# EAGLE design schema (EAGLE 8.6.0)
CNAME: Garden light controller with hysteresis; CREVISION: 4; CVERSION: V 1.0; DATECODE: 8/07/2017; DESIGNER: Michy
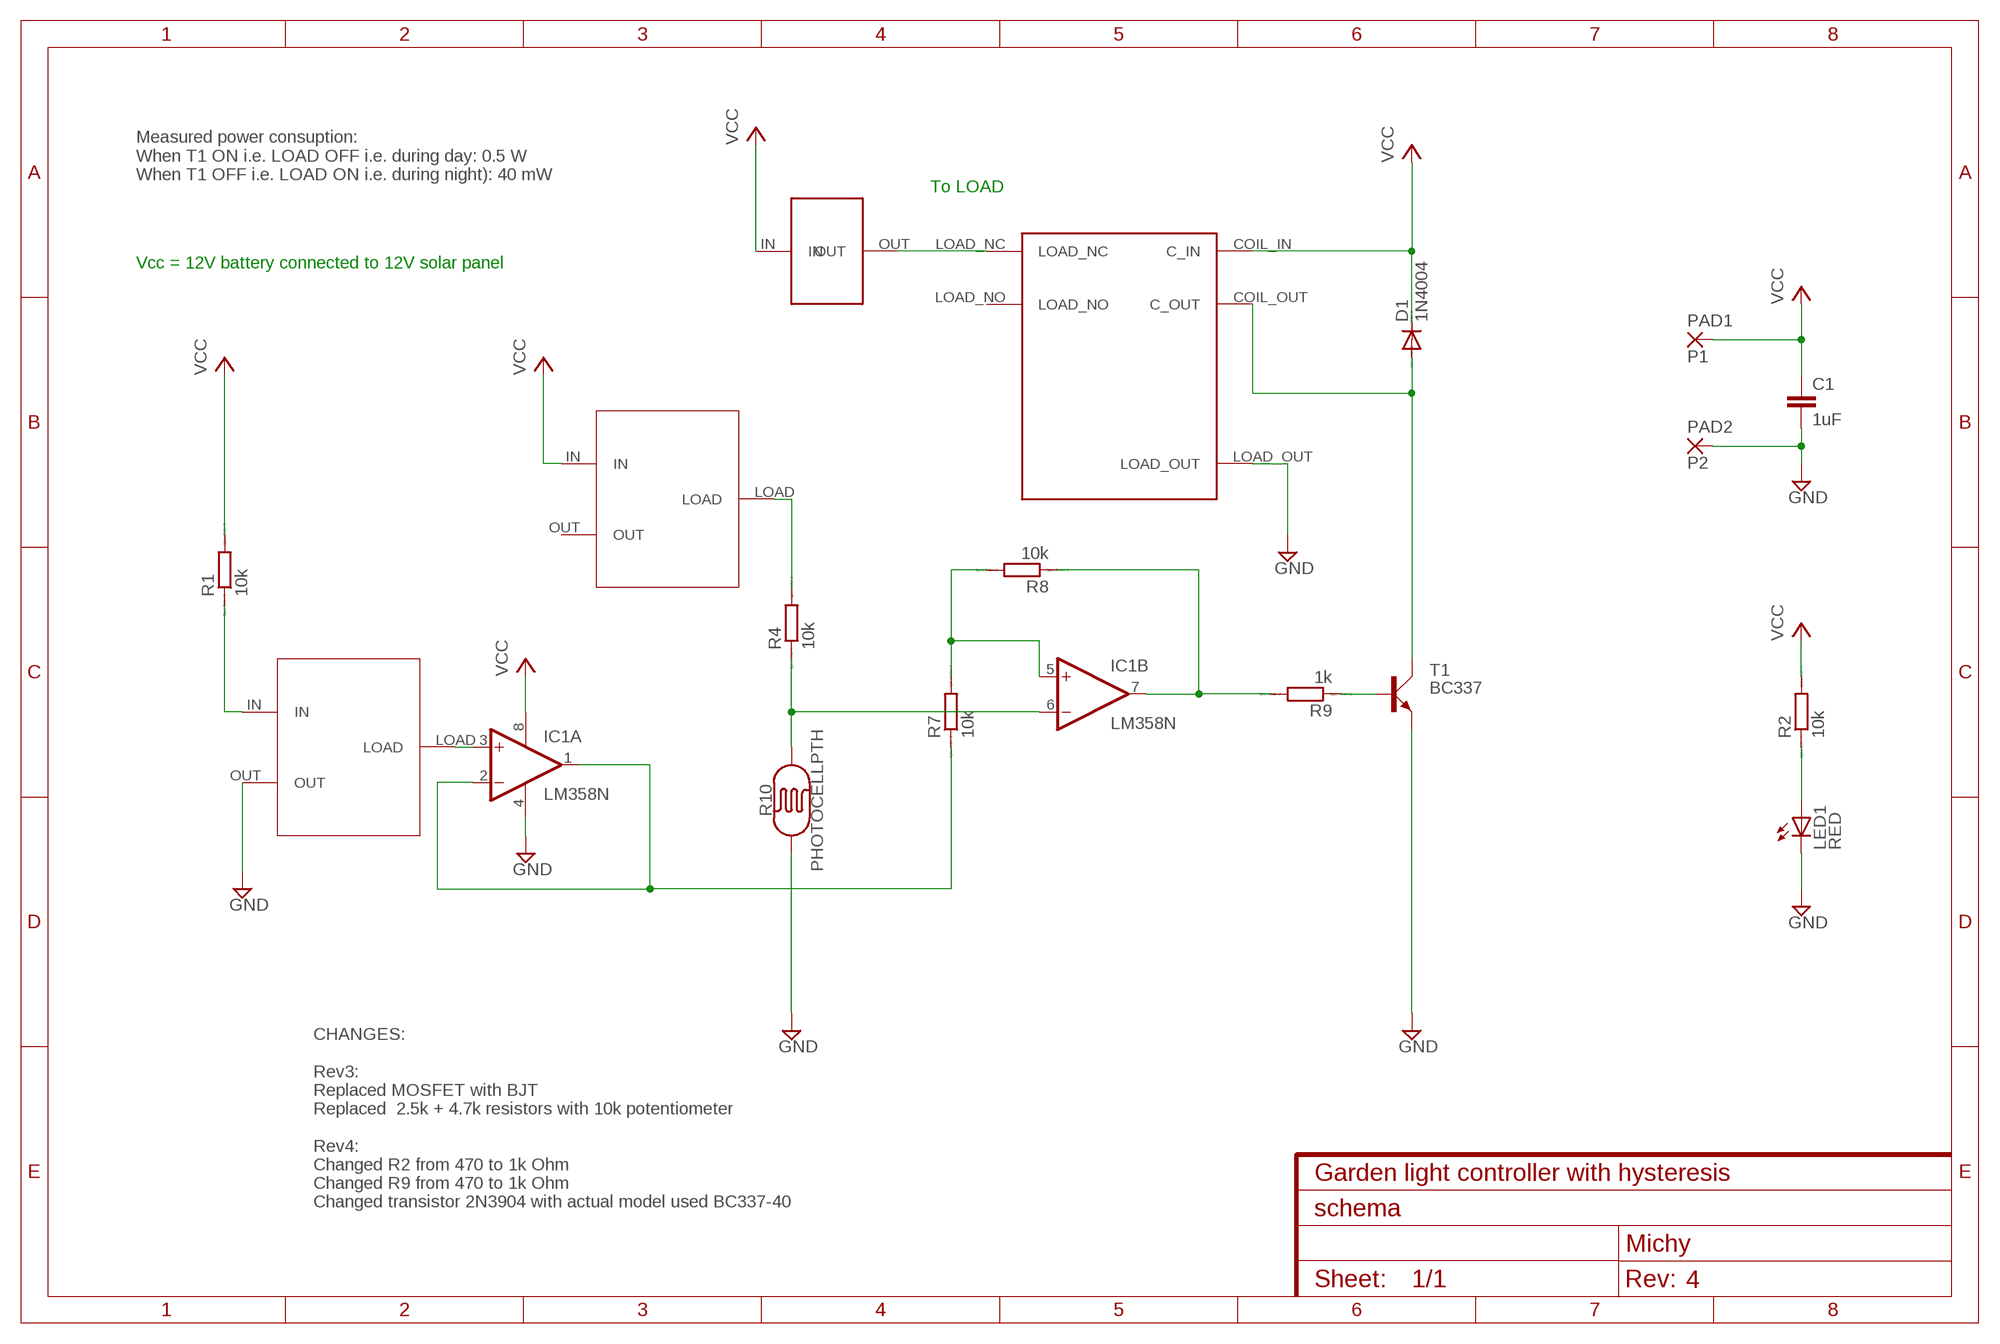
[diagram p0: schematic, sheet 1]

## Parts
C1  1uF  C-EU025-025X050  [C025-025X050]
D1  1N4004  [DO41-10]
IC1  LM358N  [DIL08]
LED1  RED  LED3MM  [LED3MM]
PAD1  P1  1,6/0,8  [1,6/0,8]
PAD2  P2  1,6/0,8  [1,6/0,8]
R1  10k  R0207/10  [0207/10]
R2  10k  R0207/10  [0207/10]
R4  10k  R0207/10  [0207/10]
R7  10k  R0207/10  [0207/10]
R8  10k  R0207/10  [0207/10]
R9  1k  R0207/10  [0207/10]
R10  PHOTOCELLPTH  [PHOTOCELL]
T1  BC337  [SOT54A]
U$1  SRSZ-12VDC-SL  [SRSZ-12VDC-SL]
U$2  ACPSPAIN22K  [ACPSPAIN22K]
U$3  ACPSPAIN22K  [ACPSPAIN22K]
U$4  DEVICEOUTLET  [OUTLET]

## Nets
GND: C1.2 IC1.4(P:V-) LED1.K(C) PAD2.1(P) R10.1 T1.E U$1.LOAD_OUT U$2.OUT
N$1: R1.1 U$2.IN
N$2: IC1.1(A:OUT) IC1.2(A:-IN) R7.1
N$3: R9.1 T1.B
N$4: LED1.A R2.1
N$5: IC1.6(B:-IN) R4.1 R10.2
N$6: R4.2 U$3.LOAD
N$7: IC1.7(B:OUT) R8.1 R9.2
N$8: IC1.5(B:+IN) R7.2 R8.2
N$9: D1.A T1.C U$1.COIL_OUT(C_OUT)
N$10: IC1.3(A:+IN) U$2.LOAD
N$11: U$1.LOAD_NC U$4.OUT
VCC: C1.1 D1.C IC1.8(P:V+) PAD1.1(P) R1.2 R2.2 U$1.COIL_IN(C_IN) U$3.IN U$4.IN
Unconnected: U$1.LOAD_NO U$3.OUT

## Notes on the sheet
- Measured power consuption:
  When T1 ON i.e. LOAD OFF i.e. during day: 0.5 W
  When T1 OFF i.e. LOAD ON i.e. during night): 40 mW
- To LOAD
- Vcc = 12V battery connected to 12V solar panel
- CHANGES:
  
  Rev3:
  Replaced MOSFET with BJT
  Replaced  2.5k + 4.7k resistors with 10k potentiometer
  
  Rev4:
  Changed R2 from 470 to 1k Ohm
  Changed R9 from 470 to 1k Ohm
  Changed transistor 2N3904 with actual model used BC337-40

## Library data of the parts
C1 = resistor:C-EU: CAPACITOR, European symbol
D1 = diode:1N4004: DIODE
IC1 = linear:LM358: OP AMP also LM158; LM258; LM2904 Source: http://cache.national.com/ds/LM/LM158.pdf
LED1 = led:LED: LED
PAD1 PAD2 = wirepad:1,6/0,8: THROUGH-HOLE PAD
R1 R2 R4 R7-R9 = eagle-ltspice:R: RESISTOR, European symbol; SPICEMODEL: NONE; SPICEPREFIX: R
R10 = SparkFun-Sensors:PHOTOCELL: Photocell (Photodetector, Photo Resistor, CdS); PROD_ID: COMP-09129; SF_ID: SEN-09088
T1 = transistor-small-signal:BC337: NPN TRANSISTOR
U$1 = custom_parts:SRSZ-12VDC-SL: SRSZ-12VDC-SL Relay
U$2 U$3 = custom_parts:ACPSPAIN22K: ACP SPAIN 22k Potentiometer
U$4 = custom_parts:DEVICEOUTLET: Device Outlet

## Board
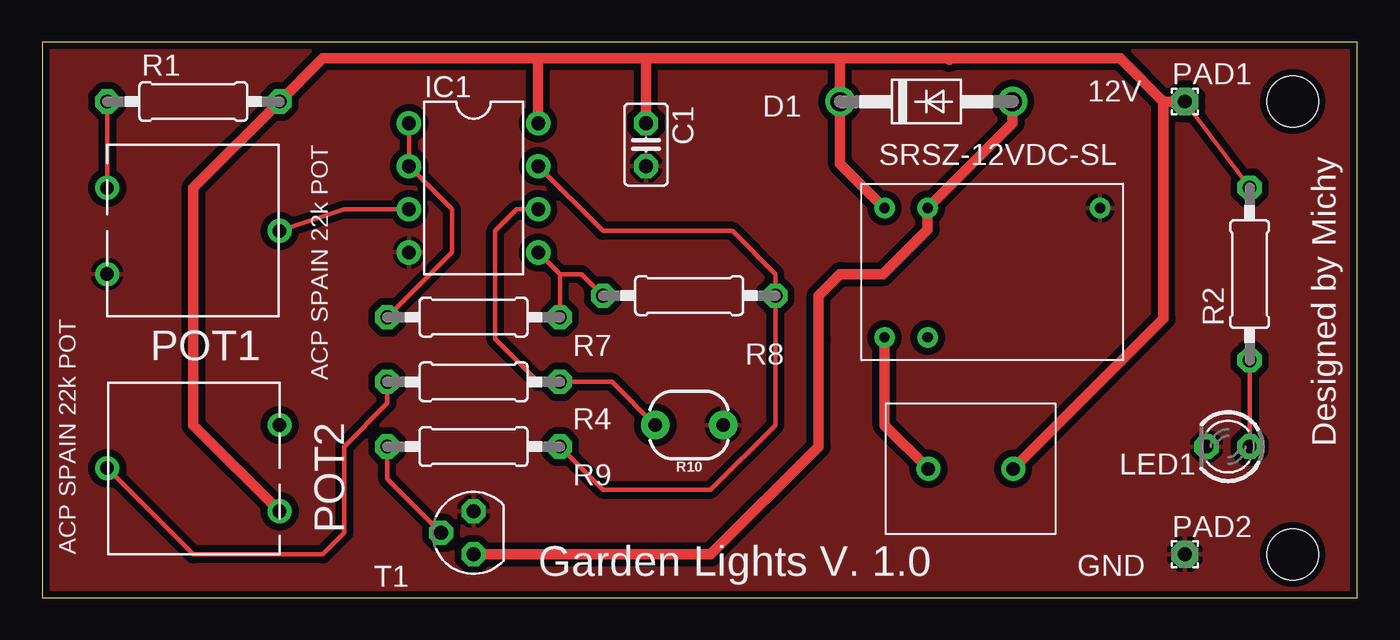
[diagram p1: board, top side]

Size 77.45 x 32.69 mm. Coordinates in mm from the lower left corner, seen from the top.
Outline: 0,0 77.45,0 77.45,32.69 0,32.69 0,0
Copper layers (1*16): Top 0.035mm / dielectric 1.5mm / Bottom 0.035mm
Design rules "SparkFun *": minimum track width 8mil, minimum drill 20mil, track to track 5mil, track to pad 5mil, pad to pad 5mil, via to via 5mil, smd to smd 5mil, copper to edge 5mil, drill to drill 5mil, minimum pad ring 12mil, minimum via ring 10mil, stop-mask expansion 4mil, vias tented up to drill 20mil, thermal gap 10mil
Holes 3 mm at 73.66,29.21 73.66,2.54

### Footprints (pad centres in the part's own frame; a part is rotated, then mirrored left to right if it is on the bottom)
C025-025X050 = drill 0.813 octagon: 1 -1.27,0; 2 1.27,0
DO41-10 = drill 1.118: A 5.08,0; C -5.08,0
DIL08 = drill 0.813 pad 1.27: 1 -3.81,-3.81; 2 -1.27,-3.81; 3 1.27,-3.81; 4 3.81,-3.81; 5 3.81,3.81; 6 1.27,3.81; 7 -1.27,3.81; 8 -3.81,3.81
LED3MM = drill 0.813 octagon: A -1.27,0; K 1.27,0
1,6/0,8 = drill 0.813 pad 1.6 octagon: 1 0,0
0207/10 = drill 0.813 octagon: 1 -5.08,0; 2 5.08,0
PHOTOCELL = drill 0.8 pad 1.676: 1 -2,0; 2 2,0
SOT54A = drill 0.813 octagon: B 0,1.905; C -1.27,0; E 1.27,0
SRSZ-12VDC-SL = drill 0.6: COIL_IN 1.35,8.97; COIL_OUT 3.89,8.97; LOAD_NC 1.35,1.35; LOAD_NO 3.89,1.35; LOAD_OUT 14.05,8.97
ACPSPAIN22K = drill 0.8: IN 2.54,0; LOAD 5.08,10.16; OUT 7.62,0
OUTLET = drill 0.8: IN 2.5,3.85; OUT 7.5,3.85

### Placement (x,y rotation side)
C1  35.56,26.67 270 top
D1  52.07,29.21 0 top
IC1  25.4,24.13 270 top
LED1  69.85,8.89 180 top
PAD1  67.31,29.21 0 top
PAD2  67.31,2.54 0 top
R1  8.89,29.21 0 top
R2  71.12,19.05 90 top
R4  25.4,12.7 180 top
R7  25.4,16.51 0 top
R8  38.1,17.78 180 top
R9  25.4,8.89 0 top
R10  38.1,10.16 180 top
T1  25.4,3.81 90 top
U$1  48.26,13.97 0 top
U$2  3.81,26.67 270 top
U$3  13.97,2.54 90 top
U$4  59.69,11.43 180 top

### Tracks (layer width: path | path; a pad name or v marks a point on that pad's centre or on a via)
GND
  pour Top (isolate 0.406): 0,0 0,33.02 77.47,33.02 77.47,0
N$1
  Top 0.254: R1.1 U$2.IN
N$2
  Top 0.254: R7.1 24.13,20.32 24.13,22.86 IC1.2 IC1.1
N$3
  Top 0.254: T1.B 20.32,6.99 R9.1
N$4
  Top 0.254: R2.1 LED1.A
N$5
  Top 0.254: IC1.6 27.94,22.86 26.67,21.59 26.67,15.24 29.21,12.7 R4.1 33.56,12.7 R10.2
N$6
  Top 0.254: R4.2 20.32,11.43 17.78,8.89 17.78,3.81 16.51,2.54 8.89,2.54 U$3.LOAD
N$7
  Top 0.254: R9.2 33.02,6.35 39.37,6.35 43.18,10.16 R8.1 43.18,19.05 40.64,21.59 33.02,21.59 IC1.7
N$8
  Top 0.254: R8.2 31.75,19.05 30.48,19.05 | 30.48,19.05 IC1.5 | R7.2 30.48,19.05
N$9
  Top 0.61: T1.C 39.37,2.54 45.72,8.89 45.72,15.24 45.72,17.78 46.99,19.05 49.53,19.05 52.15,21.67 U$1.COIL_OUT 57.15,27.94 D1.A
N$10
  Top 0.254: U$2.LOAD 17.78,22.86 IC1.3
N$11
  Top 0.61: U$4.OUT 49.61,10.16 U$1.LOAD_NC
VCC
  Top 0.254: R2.2 PAD1.1
  Top 0.61: PAD1.1 66.04,29.21 | 53.34,31.75 63.5,31.75 66.04,29.21 | 53.34,31.75 46.99,31.75 | 46.99,31.75 35.56,31.75 | 35.56,31.75 29.21,31.75 | 29.21,31.75 16.51,31.75 R1.2 8.89,24.13 8.89,10.16 U$3.IN | 53.42,31.67 53.34,31.75 | IC1.8 29.21,31.75 | U$4.IN 66.04,16.43 66.04,29.21 | C1.1 35.56,31.75 | 46.99,31.75 D1.C 46.99,25.56 U$1.COIL_IN

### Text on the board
tPlace: 12V | POT1 | Designed by Michy | POT2 | Garden Lights V. 1.0 | GND
tDocu: Design rule check: / - Default / - SparkFun

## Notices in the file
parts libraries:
SparkFun-Sensors: Licensing: Creative Commons ShareAlike 4.0 International - https://creativecommons.org/licenses/by-sa/4.0
